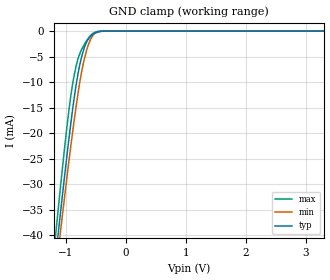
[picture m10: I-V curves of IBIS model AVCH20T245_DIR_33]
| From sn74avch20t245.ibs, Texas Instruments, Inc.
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[Model]   AVCH20T245_DIR_33
Model_type  Input
Vinl=0.8
Vinh=2.0
| variable   typ   min   max
C_comp   2.57pF   1.97pF   3.30pF
[Temperature Range]   40   100   -40
| Ambient temperature   25   85   -40
[Voltage range]   3.3   3   3.6
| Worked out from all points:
|   GND clamp passes 1 mA (typ) near -0.58 V on its own axis
[GND Clamp]
| AVCH20T245_DIR_33
|   Voltage   I(typ)   I(min)   I(max)
-4.6V     -459.2mA   -437.9mA   -484.2mA
-1.19V    -46.52mA   -49.58mA   -42.3mA
-1.16V    -43.23mA   -46.49mA   -38.76mA
-1.13V    -39.97mA   -43.42mA   -35.25mA
-1.105V   -37.28mA   -40.88mA   -32.35mA
-1.08V    -34.61mA   -38.36mA   -29.5mA
-950mV    -21.28mA   -25.63mA   -15.65mA
-835mV    -11.06mA   -15.29mA   -7.217mA
-760mV    -6.238mA   -9.522mA   -4.207mA
-680mV    -2.88mA    -4.916mA   -2.377mA
-520mV    -424.9uA   -517.7uA   -253uA
3.3V      197.1pA    969.9pA    49.62pA
